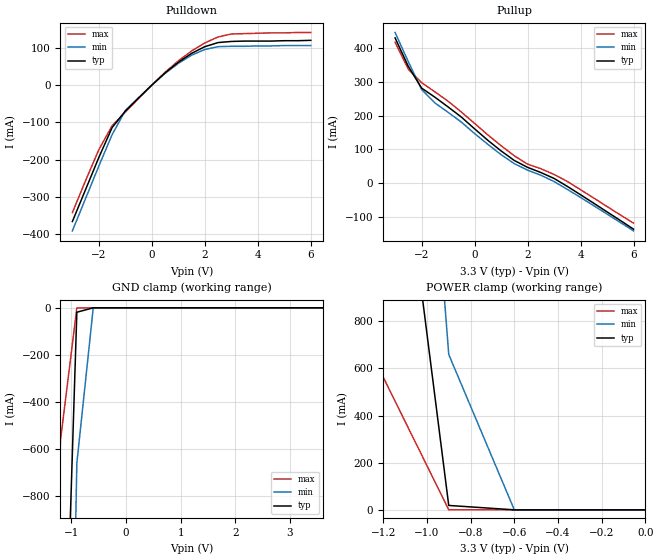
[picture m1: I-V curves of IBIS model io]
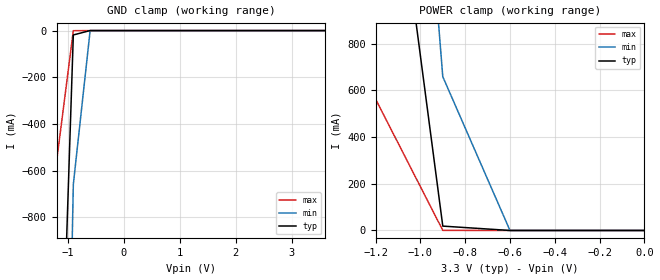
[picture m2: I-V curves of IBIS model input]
[IBIS Ver]		1.1
[File Name]	69618c.ibs
[File Rev]		1.0
[Date]		7/29/98
[Source]		File originated at Motorola
[Notes]		This file is valid for 'F' and 'P' (BurstRAM) versions of
|			the 64Kx18 FSRAM.
[Disclaimer]	This information is for modeling purposes only and
|			is not guaranteed.
[Component]	64Kx18 FSRAM
[Manufacturer]	Motorola
[Package]
|		typ		min		max
R_pkg		200m		150m		250m
L_pkg		5.5nH		4nH		7nH
C_pkg		2pF		1.5pF		2.5pF
[Pin]		signal_name	model_name		R_pin		L_pin		C_pin
1		NC			NC		NA		NA		NA
2		NC			NC		NA		NA		NA
3		NC			NC		NA		NA		NA
4		VCC			POWER		NA		NA		NA
5		VSS			GND		NA		NA		NA
6		NC			NC		NA		NA		NA
7		NC			NC		NA		NA		NA
8		DQb			io		NA		NA		NA
9		DQb			io		NA		NA		NA
10		VSS			GND		NA		NA		NA
11		VCC			POWER		NA		NA		NA
12		DQb			io		NA		NA		NA
13		DQb			io		NA		NA		NA
14		NC			NC		NA		NA		NA
15		VCC			POWER		NA		NA		NA
16		NC			NC		NA		NA		NA
17		VSS			GND		NA		NA		NA
18		DQb			io		NA		NA		NA
19		DQb			io		NA		NA		NA
20		VCC			POWER		NA		NA		NA
21		VSS			GND		NA		NA		NA
22		DQb			io		NA		NA		NA
23		DQb			io		NA		NA		NA
24		DQb			io		NA		NA		NA
25		NC			NC		NA		NA		NA
26		VSS			GND		NA		NA		NA
27		VCC			POWER		NA		NA		NA
28		NC			NC		NA		NA		NA
29		NC			NC		NA		NA		NA
30		NC			NC		NA		NA		NA
31		LBO#			NC		NA		NA		NA
32		SA			input		NA		NA		NA
33		SA			input		NA		NA		NA
34		SA			input		NA		NA		NA
35		SA			input		NA		NA		NA
36		SA1			input		NA		NA		NA
37		SA0			input		NA		NA		NA
38		NC			NC		NA		NA		NA
39		NC			NC		NA		NA		NA
40		VSS			GND		NA		NA		NA
41		VCC			POWER		NA		NA		NA
42		NC			NC		NA		NA		NA
43		NC			NC		NA		NA		NA
44		SA			input		NA		NA		NA
45		SA			input		NA		NA		NA
46		SA			input		NA		NA		NA
47		SA			input		NA		NA		NA
48		SA			input		NA		NA		NA
49		NC			NC		NA		NA		NA
50		NC			NC		NA		NA		NA
51		NC			NC		NA		NA		NA
52		NC			NC		NA		NA		NA
53		NC			NC		NA		NA		NA
54		VCC			POWER		NA		NA		NA
55		VSS			GND		NA		NA		NA
56		NC			NC		NA		NA		NA
57		NC			NC		NA		NA		NA
58		DQa			io		NA		NA		NA
59		DQa			io		NA		NA		NA
60		VSS			GND		NA		NA		NA
61		VCC			POWER		NA		NA		NA
62		DQa			io		NA		NA		NA
63		DQa			io		NA		NA		NA
64		NC			NC		NA		NA		NA
65		VCC			POWER		NA		NA		NA
66		NC			NC		NA		NA		NA
67		VSS			GND		NA		NA		NA
68		DQa			io		NA		NA		NA
69		DQa			io		NA		NA		NA
70		VCC			POWER		NA		NA		NA
71		VSS			GND		NA		NA		NA
72		DQa			io		NA		NA		NA
73		DQa			io		NA		NA		NA
74		DQa			io		NA		NA		NA
75		NC			NC		NA		NA		NA
76		VSS			GND		NA		NA		NA
77		VCC			POWER		NA		NA		NA
78		NC			NC		NA		NA		NA
79		NC			NC		NA		NA		NA
80		SA			input		NA		NA		NA
81		SA			input		NA		NA		NA
82		SA			input		NA		NA		NA
83		ADV#			input		NA		NA		NA
84		ADSP#			input		NA		NA		NA
85		ADSC#			input		NA		NA		NA
86		G#			input		NA		NA		NA
87		SW#			input		NA		NA		NA
88		SGW#			input		NA		NA		NA
89		K			input		NA		NA		NA
90		VSS			GND		NA		NA		NA
91		VCC			POWER		NA		NA		NA
92		SE3#			input		NA		NA		NA
93		SBa#			input		NA		NA		NA
94		SBb#			input		NA		NA		NA
95		NC			NC		NA		NA		NA
96		NC			NC		NA		NA		NA
97		SE2			input		NA		NA		NA
98		SE1#			input		NA		NA		NA
99		SA			input		NA		NA		NA
100		SA			input		NA		NA		NA
| Models and submodels in the file (2): io (I/O), input (Input)
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| Bi-directional IO model
[Model]	io
Model_type	I/O
Polarity	Non-Inverting
Enable	Active-Low
|signals 	DQa, DQb
|   typ		min		max
C_comp			6pF		5pF		7pF
|   typ		min		max
[Voltage range]		3.3V		3.1V		3.6V
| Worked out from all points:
|   slope of the pulldown table from 0 to 0.495 V, typ, clamps not added: 15.3 ohm
|   slope of the pullup table from 0 to 0.495 V, typ, clamps not added: 14.7 ohm
|Temperature		50C		0C		100C
|VOH   IOH
|   (mA)
|		typ		min		max
[Pullup]
-3V       431mA      447mA      418mA
-2.5V     346mA      360mA      338mA
-2V       282mA      278mA      298mA
-1.5V     255mA      238mA      271mA
-1V       226mA      210mA      243mA
-500mV    196mA      181mA      211mA
1V        95.4mA     84.3mA     111mA
1.5V      67mA       57.6mA     80.8mA
2V        46.6mA     38.3mA     56.1mA
3V        13.7mA     4.53mA     25.5mA
3.5V      -9.87mA    -18.8mA    4.86mA
6V        -137mA     -142mA     -119mA
|VOL   IOL
|   (mA)
|		typ		min		max
[Pulldown]
-3V       -366mA     -391mA     -342mA
-2V       -194mA     -217mA     -173mA
-1.5V     -114mA     -133mA     -109mA
-1V       -69.8mA    -68mA      -72.4mA
0V        -28.2pA    -21.3pA    -27nA
500mV     32.6mA     31.3mA     34.3mA
1V        61.1mA     58.3mA     64.9mA
1.5V      85mA       80.1mA     91.4mA
2V        103mA      95.5mA     113mA
2.5V      114mA      103mA      129mA
3V        117mA      104mA      137mA
6V        120mA      106mA      141mA
|Voltage
|		typ		min		max
[GND_clamp]
-3.6V     -35A       -37.4A     -32.6A
-1.5V     -6.04A     -8.28A     -3.9A
-1.2V     -2.21A     -4.26A     -563mA
-900mV    -18.8mA    -659mA     -562uA
-600mV    -101uA     -143uA     -100uA
3.6V      -100uA     -100uA     -100uA
|Voltage
|		typ		min		max
[POWER_clamp]
-3.6V     35A        37.4A      32.6A
-1.5V     6.04A      8.28A      3.9A
-1.2V     2.21A      4.26A      563mA
-900mV    18.8mA     659mA      562uA
-600mV    101uA      143uA      100uA
0V        100uA      100uA      100uA
[Ramp]
|variable	typ		min		max
dV/dt_r	1.9/2.0n	1.7/2.4n	2.3/1.6n
dV/dt_f	2.4/1.5n	2.0/1.8n	2.6/1.2n
| Standard Input model
[Model]		input
Model_type		Input
Polarity		Non-Inverting
|signals  SA, K, ADSP#, ADSC#, ADV#, SBa#, SBb#,
|			SE1#, SE2, SE3#, SW#, SGW#, G#
Vinl = 0.8V
Vinh = 2.0V
|   typ		min		max
C_comp			3.5pF		3pF		4pF
|   typ		min		max
[Voltage range]		3.3V		3.1V		3.6V
|Temperature		50C		0C		100C
[GND_clamp]
|Voltage	I(typ)	I(min)	I(max)
-3.6V     -35A       -37.4A     -32.6A
-1.5V     -6.04A     -8.28A     -3.9A
-1.2V     -2.21A     -4.26A     -563mA
-900mV    -18.8mA    -659mA     -562uA
-600mV    -101uA     -143uA     -100uA
3.6V      -100uA     -100uA     -100uA
[POWER_clamp]
|Voltage	I(typ)	I(min)	I(max)
-3.6V     35A        37.4A      32.6A
-1.5V     6.04A      8.28A      3.9A
-1.2V     2.21A      4.26A      563mA
-900mV    18.8mA     659mA      562uA
-600mV    101uA      143uA      100uA
0V        100uA      100uA      100uA
